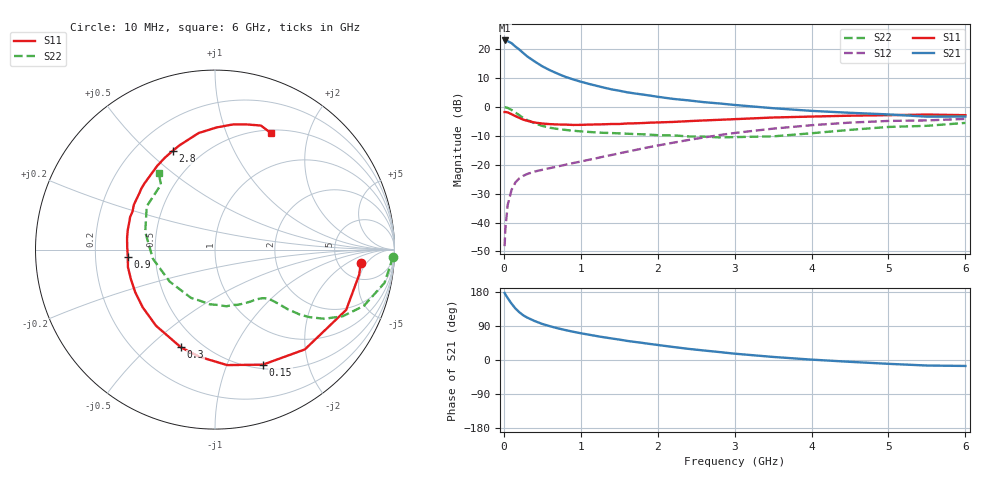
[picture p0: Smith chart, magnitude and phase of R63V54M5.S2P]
! SIEMENS Small Signal Semiconductors
! BFR193
! Si NPN RF Bipolar Junction Transistor in SOT23
! VCE = 3.5 V  IC = 4.5 mA
! Common Emitter S-Parameters:  May  1996
# GHz  S  MA  R  50
!  f  S11  S21  S12  S22
! GHz  MAG  ANG  MAG  ANG  MAG  ANG  MAG  ANG
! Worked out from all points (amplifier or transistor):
!   36 points, 10 MHz to 6 GHz, reference 50 ohm
!   highest |S21| = 23.0 dB at 10 MHz (marker M1)
!   |S21| within 3 dB of that: start of sweep to 194.3 MHz
!   unconditionally stable (mu >= 1): 927.9 MHz to 2.009 GHz
!   at 250 MHz: K = 0.40, MSG = 21.3 dB, |S12| = -23.9 dB
!   at 1.4 GHz: K = 1.07, MAG = 9.8 dB, |S12| = -16.6 dB
!   at 6 GHz: K = 0.97, MSG = 0.4 dB, |S12| = -4.1 dB
!   S11 on the Smith chart (normalised r, x): 10 MHz: 8.18, -3.68; 150 MHz: 0.55, -1.35; 300 MHz: 0.39, -0.64; 900 MHz: 0.35, -0.04; 2.8 GHz: 0.35, +0.60; 6 GHz: 0.54, +1.45
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0.01  0.8158 -5.3  14.11 176.8  0.0039 88.6  0.9927 -2.3
0.02  0.8154 -9.9  13.88 173.2  0.0079 84.9  0.9833 -4.5
0.05  0.8043 -24.7  13.71 163.5  0.0201 77.9  0.9626 -11.1
0.1  0.7483 -48.0  12.68 148.8  0.0367 67.2  0.8867 -20.7
0.15  0.6943 -67.4  11.07 136.1  0.0493 59.3  0.8022 -27.6
0.2  0.647 -84.0  9.862 126.3  0.058 53.6  0.721 -32.3
0.25  0.6035 -98.3  8.62 118.3  0.064 49.6  0.6488 -35.5
0.3  0.5768 -109.2  7.553 112.3  0.0688 47.9  0.5969 -37.4
0.4  0.5366 -127.8  6.115 102.9  0.0762 45.5  0.5219 -39.4
0.5  0.5155 -141.4  5.043 95.1  0.0817 45.8  0.469 -40.4
0.6  0.5038 -152.0  4.306 89.1  0.0874 47.1  0.436 -41.3
0.7  0.4967 -160.7  3.756 83.7  0.0934 48.1  0.4158 -42.1
0.9  0.4875 -175.3  2.993 74.6  0.1067 51.1  0.3878 -44.3
1.1  0.4939 172.7  2.512 67.0  0.1213 54.6  0.3693 -47.8
1.3  0.5005 163.3  2.158 60.0  0.1385 56.7  0.356 -51.8
1.6  0.5167 151.0  1.793 50.5  0.1677 58.7  0.3441 -59.4
2.2  0.5497 130.6  1.377 34.4  0.2401 57.8  0.3221 -78.7
2.8  0.5982 113.3  1.148 21.0  0.325 51.8  0.297 -105.9
3.5  0.6558 98.0  0.95 8.1  0.4208 41.2  0.3094 -144.9
4.5  0.705 81.7  0.791 -4.8  0.5354 23.9  0.4009 165.8
5.5  0.737 69.7  0.678 -14.6  0.584 6.5  0.4712 129.7
6  0.7201 64.3  0.681 -15.7  0.6209 1.5  0.5288 126.4
